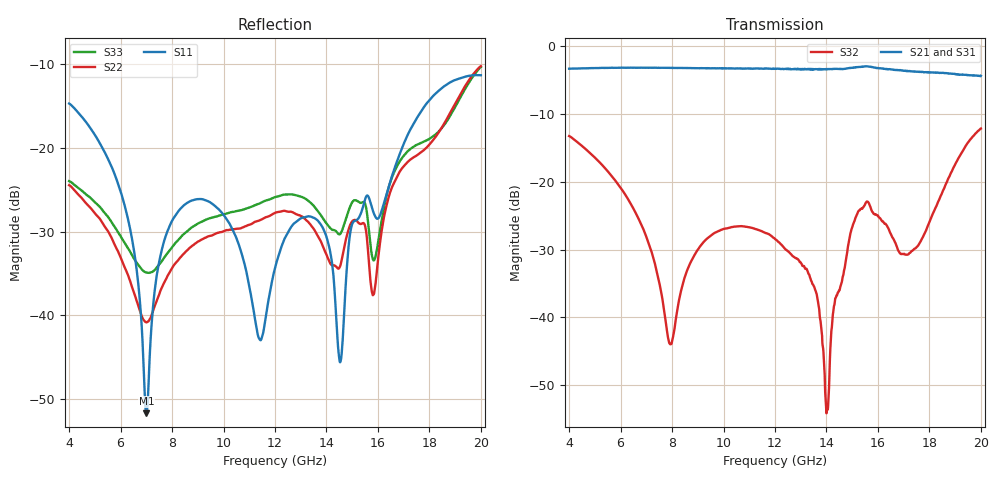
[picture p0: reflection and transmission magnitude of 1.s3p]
!The following data was pulled from an Agilent PNA
!This sNp file was generated from the data in the RF Test software
!NOTE:  Smoothing/Math/Corrections applied on any given trace ARE included in the data saved here
# MHz S dB R 50
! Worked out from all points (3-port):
!   1601 points, 4 GHz to 20 GHz, reference 50 ohm
!   strongest paths, dB at 4 GHz, 8 GHz, 12 GHz, 16 GHz, 20 GHz:
!     S21: -3.3, -3.2, -3.3, -3.2, -4.3
!     S31: -3.3, -3.2, -3.3, -3.2, -4.3
!     S32: -13.2, -43.5, -28.4, -25.0, -12.1
!   lowest |S11| = -51.7 dB at 7 GHz (marker M1), VSWR 1.01, Z = 50.1 - j0.25 ohm
!   |S11| at or under -10 dB: start of sweep to end of sweep
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4000  -14.68 90.8  -3.30 -108.8  -3.29 -108.9
      -3.30 -108.7  -24.44 -55.5  -13.24 -140.2
      -3.29 -108.7  -13.24 -140.2  -23.95 -59.3
6180  -27.13 34.7  -3.15 -171.9  -3.15 -172.0
      -3.16 -172.0  -34.41 -129.9  -21.88 161.2
      -3.17 -172.0  -21.88 161.2  -31.45 -124.2
7000  -51.72 -74.4  -3.16 163.6  -3.16 163.5
      -3.15 163.6  -40.84 -98.4  -28.12 142.7
      -3.17 163.6  -28.11 142.7  -34.88 -106.6
8370  -27.11 160.3  -3.18 121.9  -3.18 121.8
      -3.18 121.9  -32.91 -66.6  -35.78 -110.5
      -3.18 121.8  -35.76 -110.5  -30.54 -79.8
12000  -34.36 -108.5  -3.29 4.4  -3.30 4.3
       -3.31 4.7  -27.75 -86.5  -28.41 167.5
       -3.30 4.6  -28.42 167.5  -25.87 -92.2
14020  -30.81 142.2  -3.35 -66.6  -3.35 -66.5
       -3.34 -66.7  -32.90 -104.5  -53.35 -155.1
       -3.38 -66.6  -53.62 -157.9  -29.10 -106.5
14530  -45.62 53.7  -3.32 -85.6  -3.32 -85.5
       -3.34 -85.6  -34.13 -69.3  -35.59 -106.0
       -3.34 -85.4  -35.63 -105.8  -30.29 -87.0
15190  -28.57 -133.8  -3.08 -111.2  -3.01 -111.5
       -3.07 -111.2  -28.75 -80.2  -24.78 -127.7
       -3.00 -111.5  -24.78 -127.6  -26.32 -89.8
16820  -20.93 -37.3  -3.48 179.2  -3.48 179.1
       -3.53 179.3  -22.97 -65.5  -30.27 167.7
       -3.57 179.1  -30.31 167.3  -21.72 -72.5
20000  -11.29 163.7  -4.56 39.2  -4.50 38.4
       -4.34 38.6  -10.21 34.2  -12.08 157.9
       -4.32 37.9  -12.12 158.2  -10.31 33.6
